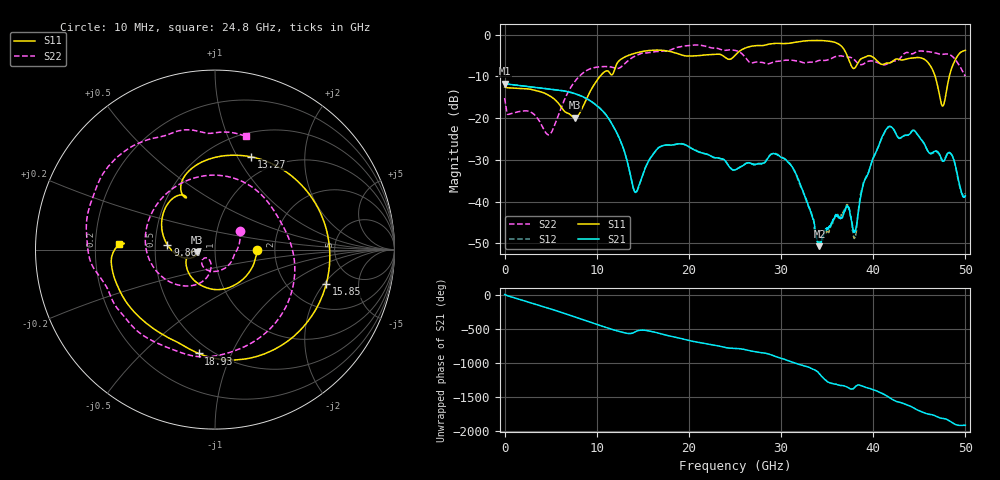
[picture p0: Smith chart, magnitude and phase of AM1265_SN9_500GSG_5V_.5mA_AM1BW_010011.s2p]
!Keysight Technologies,N5245B,MY58422270,A.16.20.02
!Date: Thursday, March 05, 2026 00:54:49
!Correction: S11(C  2-Port  )
!S21(C  2-Port  )
!S12(C  2-Port  )
!S22(C  2-Port  )
!S2P File: Measurements: S11, S21, S12, S22:
# Hz S  dB  R 50
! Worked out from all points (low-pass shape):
!   3201 points, 10 MHz to 50 GHz, reference 50 ohm
!   highest |S21| = -11.76 dB at 10 MHz (marker M1); lowest = -50.7 dB at 34.16 GHz (marker M2)
!   |S21| within 3 dB of the highest: start of sweep to 8.383 GHz
!   lowest |S11| = -19.9 dB at 7.633 GHz (marker M3), VSWR 1.22, Z = 40.9 - j1.29 ohm
!   |S11| at or under -10 dB: start of sweep to 10.35 GHz; 46.72 GHz to 48.25 GHz (1.537 GHz wide, 3.24 % of centre)
!   |S22| runs from -24.0 to -2.5 dB; largest |S21 - S12| = 0.0059
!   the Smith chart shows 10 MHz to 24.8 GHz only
!   S11 on the Smith chart (normalised r, x): 10 MHz: 1.62, -0.01; 9.867 GHz: 0.58, +0.03; 13.27 GHz: 0.77, +1.15; 15.85 GHz: 3.19, -2.12; 18.93 GHz: 0.43, -0.76; 24.8 GHz: 0.30, +0.03
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1e7  -12.53 -0.4  -11.76 4.1  -11.81 2.8  -15.18 37.1
4.821538e9  -14.54 -147.2  -13.01 160.9  -13.02 161.0  -24.01 -124.8
7.633475e9  -19.92 -171.1  -14.13 36.0  -14.12 36.1  -11.22 -133.2
8.352081e9  -17.98 -160.6  -14.73 2.9  -14.72 3.0  -9.48 -154.6
9.867403e9  -11.48 174.2  -16.75 -66.7  -16.73 -66.8  -7.83 152.4
1.146083e10  -9.35 118.9  -20.69 -139.2  -20.68 -139.2  -7.70 76.8
1.327297e10  -5.11 68.5  -30.04 155.8  -30.05 156.3  -6.49 -21.8
1.424153e10  -4.38 34.7  -37.81 -178.1  -37.82 -178.1  -5.04 -69.3
1.585058e10  -3.76 -17.2  -29.48 -174.7  -29.47 -174.7  -4.22 -123.4
1.667854e10  -3.69 -42.1  -27.13 159.1  -27.16 159.0  -4.04 -143.1
1.892809e10  -4.65 -99.0  -26.15 86.3  -26.12 86.2  -2.95 177.7
2.480192e10  -5.42 176.6  -32.42 -63.7  -32.41 -63.4  -3.68 74.8
2.5005e10  -4.96 175.3  -32.40 -64.5  -32.40 -63.6  -3.76 70.2
2.951972e10  -2.06 96.4  -28.69 171.1  -28.57 170.6  -6.39 -18.0
3.334708e10  -1.41 35.7  -43.29 -4.1  -43.22 -0.1  -6.59 -132.8
3.415942e10  -1.38 21.6  -50.69 -79.3  -49.45 -67.8  -6.16 -150.3
3.712758e10  -4.76 -40.2  -41.23 90.9  -40.73 88.1  -5.33 151.1
3.80024e10  -7.98 -26.8  -46.99 84.9  -48.67 86.6  -6.11 134.1
4.167354e10  -6.78 -54.6  -22.05 -59.9  -22.13 -59.8  -6.83 112.4
4.518846e10  -5.56 -102.1  -25.04 88.5  -25.09 89.1  -3.90 73.7
4.770358e10  -16.35 70.5  -30.18 -14.7  -29.97 -14.1  -4.66 41.0
5e10  -3.74 -71.3  -38.60 -113.0  -38.05 -110.0  -9.94 8.1
